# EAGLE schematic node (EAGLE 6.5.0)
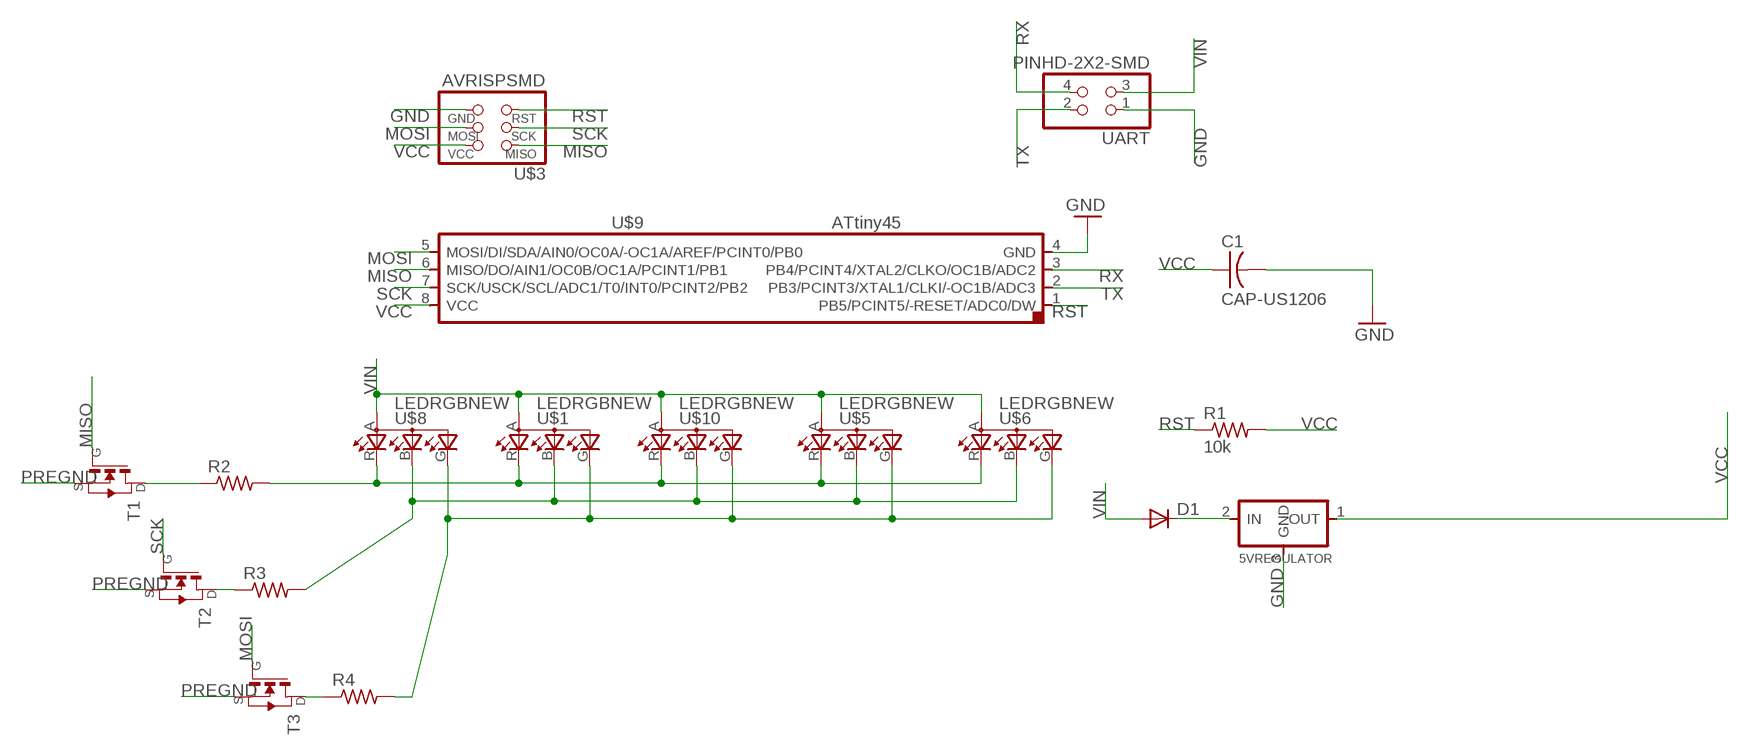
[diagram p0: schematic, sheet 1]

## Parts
5VREGULATOR  REGULATORSOT23  [SOT23]
C1  CAP-US1206  [C1206]
D1  DIODESOD123  [SOD123]
R1  10k  RES-US1206  [R1206]
R2  RES-US1206  [R1206]
R3  RES-US1206  [R1206]
R4  RES-US1206  [R1206]
T1  NMOSFETSOT23  [SOT-23]
T2  NMOSFETSOT23  [SOT-23]
T3  NMOSFETSOT23  [SOT-23]
U$1  LEDRGBNEW  [P-LCC-4]
U$3  AVRISPSMD  [2X03SMD]
U$5  LEDRGBNEW  [P-LCC-4]
U$6  LEDRGBNEW  [P-LCC-4]
U$8  LEDRGBNEW  [P-LCC-4]
U$9  ATTINY45SI  [SOIC8]
U$10  LEDRGBNEW  [P-LCC-4]
UART  PINHD-2X2-SMD  [2X02SMD]

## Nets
GND: 5VREGULATOR.3(GND) C1.2 U$3.6(GND) U$9.4(GND) UART.1
MISO: T1.3(G) U$3.1(MISO) U$9.6(MISO/DO/AIN1/OC0B/OC1A/PCINT1/PB1)
MOSI: T3.3(G) U$3.4(MOSI) U$9.5(MOSI/DI/SDA/AIN0/OC0A/-OC1A/AREF/PCINT0/PB0)
N$1: R2.2 U$1.R(CRED) U$5.R(CRED) U$6.R(CRED) U$8.R(CRED) U$10.R(CRED)
N$2: R3.2 U$1.B(CBLUE) U$5.B(CBLUE) U$6.B(CBLUE) U$8.B(CBLUE) U$10.B(CBLUE)
N$3: R4.2 U$1.G(CGREEN) U$5.G(CGREEN) U$6.G(CGREEN) U$8.G(CGREEN) U$10.G(CGREEN)
N$4: 5VREGULATOR.2(IN) D1.CATHODE(C)
N$7: R2.1 T1.1(D)
N$15: R3.1 T2.1(D)
N$16: R4.1 T3.1(D)
PREGND: T1.2(S) T2.2(S) T3.2(S)
RST: R1.1 U$3.5(RST) U$9.1(PB5/PCINT5/-RESET/ADC0/DW)
RX: U$9.3(PB4/PCINT4/XTAL2/CLKO/OC1B/ADC2) UART.4
SCK: T2.3(G) U$3.3(SCK) U$9.7(SCK/USCK/SCL/ADC1/T0/INT0/PCINT2/PB2)
TX: U$9.2(PB3/PCINT3/XTAL1/CLKI/-OC1B/ADC3) UART.2
VCC: 5VREGULATOR.1(OUT) C1.1 R1.2 U$3.2(VCC) U$9.8(VCC)
VIN: D1.ANODE(A) U$1.A(A2) U$5.A(A2) U$6.A(A2) U$8.A(A2) U$10.A(A2) UART.3

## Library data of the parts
5VREGULATOR = 01_fab:REGULATOR
C1 = fab:CAP-US
D1 = 01_fab:DIODE: DIODE
R1-R4 = fab:RES-US: Resistor (US Symbol)
T1-T3 = fab:NMOSFET: MOS FET
U$1 U$5 U$6 U$8 U$10 = Juanes Library:LEDRGBNEW
U$3 = fab:AVRISP
U$9 = 01_fab:ATTINY45
UART = 01_fab:PINHD-2X2-SMD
